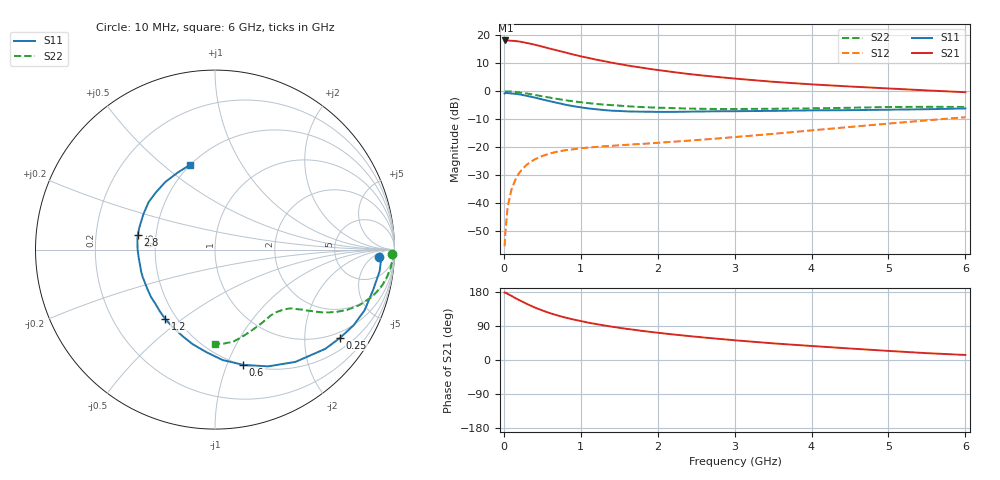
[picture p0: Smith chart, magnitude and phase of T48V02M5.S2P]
! Infineon Technologies  Discrete & RF Semiconductors
! BFR182T
! Si NPN RF Bipolar Junction Transistor in SC75
! VCE = 8 V  IC = 2.5 mA
! Common Emitter S-Parameters:  October  1999
# GHz  S  MA  R  50
!  f  S11  S21  S12  S22
! GHz  MAG  ANG  MAG  ANG  MAG  ANG  MAG  ANG
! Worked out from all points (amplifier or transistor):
!   36 points, 10 MHz to 6 GHz, reference 50 ohm
!   highest |S21| = 18.1 dB at 20 MHz (marker M1)
!   |S21| within 3 dB of that: start of sweep to 611.8 MHz
!   unconditionally stable (mu >= 1): 1.923 GHz to 4.36 GHz
!   at 250 MHz: K = 0.17, MSG = 22.5 dB, |S12| = -27.6 dB
!   at 1.4 GHz: K = 0.82, MSG = 14.9 dB, |S12| = -19.5 dB
!   at 6 GHz: K = 0.84, MSG = 4.5 dB, |S12| = -9.3 dB
!   lowest NFmin = 1.10 dB at 450 MHz
!   S11 on the Smith chart (normalised r, x): 10 MHz: 18, -9; 250 MHz: 0.82, -2.96; 600 MHz: 0.50, -1.14; 1.2 GHz: 0.43, -0.44; 2.8 GHz: 0.39, +0.08; 6 GHz: 0.50, +0.62
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0.01  0.914 -2.6  8.06 178.0  0.0017 82.0  0.9868 -1.4
0.02  0.9289 -1.6  8.075 178.0  0.003 85.1  0.9922 -1.2
0.05  0.9253 -7.4  8.067 174.3  0.0086 90.2  0.9908 -3.2
0.1  0.9094 -14.2  7.971 169.1  0.0177 82.6  0.9831 -6.2
0.15  0.8995 -22.1  7.881 163.4  0.0262 77.2  0.9692 -9.2
0.25  0.8531 -35.1  7.501 153.0  0.0417 70.8  0.9316 -14.6
0.3  0.8266 -42.0  7.275 148.0  0.0489 67.6  0.91 -17.0
0.4  0.7695 -54.4  6.792 138.7  0.0603 61.7  0.8601 -21.2
0.5  0.7146 -65.6  6.273 130.8  0.0697 57.5  0.8121 -24.3
0.6  0.6612 -76.2  5.771 123.6  0.0772 53.7  0.767 -26.8
0.8  0.5744 -94.6  4.922 111.9  0.0882 48.7  0.691 -30.4
0.9  0.5412 -103.4  4.536 107.1  0.0915 47.1  0.6596 -31.6
1.1  0.4917 -118.6  3.932 98.4  0.0984 45.2  0.6128 -33.6
1.2  0.4763 -125.4  3.669 94.9  0.1009 44.4  0.5927 -34.4
1.4  0.4487 -137.8  3.236 88.1  0.1055 44.1  0.5642 -36.0
1.6  0.4362 -149.5  2.895 82.1  0.1102 44.6  0.5394 -37.4
2.2  0.4275 -173.9  2.202 67.4  0.1251 48.2  0.4991 -42.9
2.8  0.4381 169.0  1.784 55.7  0.1437 52.4  0.4806 -49.7
3.5  0.4453 153.6  1.474 43.9  0.1728 56.3  0.4858 -58.1
4.5  0.4584 135.7  1.214 30.3  0.2298 57.9  0.5061 -71.6
5.5  0.4763 116.2  1.034 18.0  0.3017 55.9  0.5262 -84.5
6  0.4924 106.6  0.959 13.3  0.3425 53.2  0.5235 -90.2
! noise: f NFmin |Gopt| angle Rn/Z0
0.45  1.1  0.39  29  0.35
0.9  1.2  0.37  59  0.28
1.8  1.8  0.28  128  0.2
